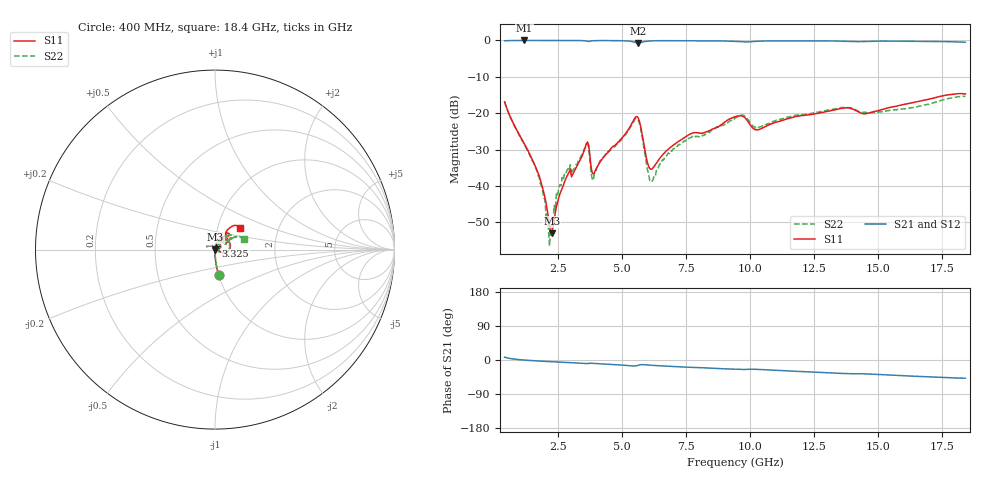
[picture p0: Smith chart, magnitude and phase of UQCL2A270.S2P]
! AVX Corporation
! Date:  10/27/06
! Part No:  UQCL2A270
! Description:  Ultra Low ESR Microwave capacitors
! Mounting Orientation:  Horizontal
# GHZ S DB R 50
! Freq  |S11|  S11 Ph  |S21|  S21 Ph  |S12|  S12 Ph  |S22|  S22 Ph
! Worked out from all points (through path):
!   401 points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, 400 MHz to 18.4 GHz, reference 50 ohm
!   highest |S21| = -0.01 dB at 1.165 GHz (marker M1); lowest = -0.8 dB at 5.62 GHz (marker M2)
!   group delay of S21, straight-line fit = 7.56 ps
!   lowest |S11| = -53.1 dB at 2.245 GHz (marker M3), VSWR 1.00, Z = 50.2 + j0.0212 ohm
!   |S11| at or under -10 dB: start of sweep to end of sweep
!   |S22| runs from -56.5 to -15.3 dB; largest |S21 - S12| = 0.0022
!   S11 on the Smith chart (normalised r, x): 400 MHz: 1.00, -0.29; 3.325 GHz: 1.01, +0.04; 18.4 GHz: 1.28, +0.32
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0.4  -16.89 -81.8  -0.11 7.4  -0.11 7.4  -16.83 -81.1
1.165  -28.37 -88.3  -0.01 -0.2  -0.02 -0.1  -28.65 -87.8
1.75  -37.23 -86.2  -0.01 -2.8  -0.02 -2.7  -37.48 -89.0
2.11  -48.59 -59.4  -0.01 -4.1  -0.01 -4.1  -51.57 -34.3
2.245  -53.06 5.4  -0.01 -4.5  -0.02 -4.5  -52.06 57.5
2.425  -45.73 61.3  -0.01 -5.2  -0.02 -5.2  -42.06 58.7
2.65  -40.70 77.3  -0.02 -6.0  -0.02 -5.9  -37.64 66.4
3.325  -33.25 74.8  -0.04 -8.3  -0.04 -8.3  -32.86 76.5
3.415  -31.94 73.2  -0.05 -8.7  -0.05 -8.7  -31.41 72.5
3.64  -27.92 41.6  -0.24 -9.5  -0.25 -9.5  -28.40 38.9
3.865  -36.74 43.8  -0.08 -8.9  -0.09 -8.9  -38.47 54.9
4.225  -32.45 70.7  -0.04 -10.4  -0.04 -10.4  -32.27 75.8
5.62  -21.31 6.7  -0.75 -14.0  -0.74 -13.9  -21.80 5.0
6.07  -35.23 9.7  -0.15 -13.5  -0.15 -13.5  -38.51 1.5
6.43  -32.68 53.4  -0.08 -15.2  -0.08 -15.1  -34.50 56.6
7.42  -26.72 63.8  -0.07 -18.6  -0.07 -18.6  -27.58 62.6
9.4  -20.99 52.7  -0.23 -24.5  -0.23 -24.4  -21.32 43.8
9.715  -20.88 38.5  -0.38 -25.1  -0.38 -25.0  -20.49 31.5
10.255  -24.57 42.7  -0.24 -24.7  -0.23 -24.6  -23.80 34.2
12.415  -20.32 54.9  -0.12 -31.7  -0.11 -31.6  -20.07 50.0
15.43  -18.44 58.0  -0.18 -39.7  -0.18 -39.7  -19.19 36.2
18.4  -14.71 40.8  -0.49 -48.0  -0.49 -48.0  -15.38 19.9
